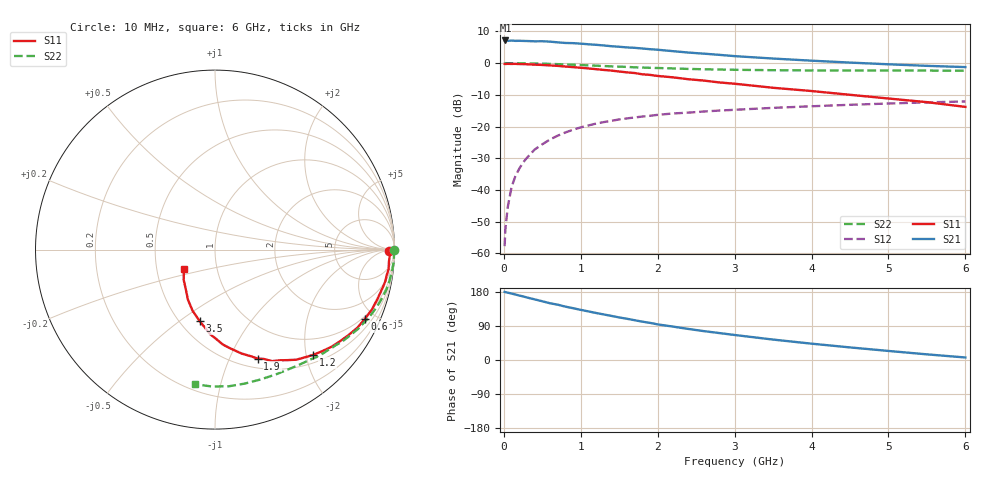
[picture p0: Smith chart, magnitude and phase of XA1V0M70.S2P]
! SIEMENS Discrete & RF Semiconductors
! BFY180
! Si NPN RF Bipolar Junction Transistor in MICRO-X
! VCE = 1 V  IC = 0.7 mA
! Common Emitter S-Parameters:  May  1997
# GHz  S  MA  R  50
!  f  S11  S21  S12  S22
! GHz  MAG  ANG  MAG  ANG  MAG  ANG  MAG  ANG
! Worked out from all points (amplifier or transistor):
!   36 points, 10 MHz to 6 GHz, reference 50 ohm
!   highest |S21| = 7.1 dB at 20 MHz (marker M1)
!   |S21| within 3 dB of that: start of sweep to 2.031 GHz
!   unconditionally stable (mu >= 1): 3.753 GHz to end of sweep
!   at 250 MHz: K = 0.08, MSG = 19.2 dB, |S12| = -31.3 dB
!   at 1.4 GHz: K = 0.49, MSG = 11.7 dB, |S12| = -18.2 dB
!   at 6 GHz: K = 1.09, MAG = 3.5 dB, |S12| = -12.1 dB
!   S11 on the Smith chart (normalised r, x): 10 MHz: 65, -16; 600 MHz: 0.87, -4.38; 1.2 GHz: 0.65, -2.14; 1.9 GHz: 0.61, -1.28; 3.5 GHz: 0.62, -0.60; 6 GHz: 0.69, -0.16
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0.01  0.9715 -0.4  2.259 179.9  0.0013 88.4  0.9973 -0.2
0.02  0.9701 -1.0  2.277 179.0  0.0024 99.5  0.9999 -0.5
0.05  0.9741 -2.0  2.243 177.8  0.0053 85.7  0.9974 -1.2
0.1  0.9714 -4.0  2.267 175.3  0.0111 87.8  0.9978 -2.6
0.15  0.9735 -6.4  2.243 172.8  0.0165 85.7  0.9981 -3.9
0.25  0.9653 -10.5  2.24 167.8  0.0271 82.8  0.9941 -6.6
0.4  0.9465 -16.7  2.209 160.0  0.0434 77.9  0.987 -10.3
0.5  0.9359 -20.9  2.213 155.0  0.0525 74.6  0.9814 -12.9
0.6  0.92 -24.8  2.181 149.7  0.0625 71.9  0.9721 -15.4
0.9  0.8646 -36.1  2.065 136.7  0.0891 63.2  0.9434 -22.4
1.1  0.8245 -43.2  1.982 128.2  0.1041 58.2  0.921 -26.8
1.2  0.8026 -46.9  1.944 124.0  0.1115 55.4  0.9116 -29.0
1.5  0.7376 -56.6  1.811 112.3  0.1294 49.2  0.8801 -34.7
1.7  0.6979 -62.9  1.743 105.0  0.139 45.6  0.859 -38.2
1.9  0.6522 -68.6  1.658 98.0  0.1479 42.2  0.843 -41.5
2.2  0.5967 -75.8  1.543 88.1  0.1608 37.6  0.8251 -46.4
2.6  0.5306 -85.3  1.41 76.2  0.1726 32.7  0.8004 -52.0
2.8  0.4961 -89.5  1.351 71.1  0.1786 30.5  0.7922 -54.8
3.5  0.4086 -101.9  1.181 53.9  0.1971 23.6  0.7737 -64.0
4.5  0.3165 -118.5  1.02 33.2  0.2203 14.8  0.7647 -77.5
5.5  0.2425 -136.0  0.906 14.9  0.2406 6.1  0.7627 -91.5
6  0.2041 -147.9  0.866 6.6  0.2487 1.7  0.7582 -98.5
